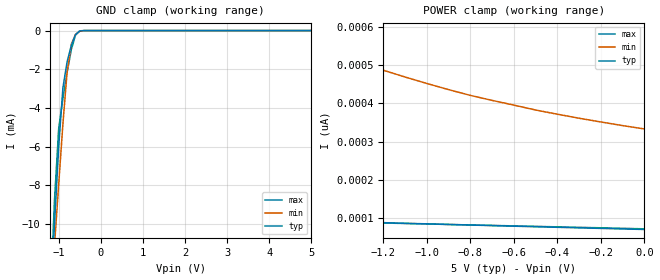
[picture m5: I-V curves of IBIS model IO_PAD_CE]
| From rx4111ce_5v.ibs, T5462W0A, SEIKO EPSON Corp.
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[Model]   IO_PAD_CE
Model_type Input
Enable Active-High
Polarity Non-Inverting
Vinh=4.4
Vinl=0.9
C_comp   2.5p   2.0p   3.0p
[Temperature Range] 25   105   -40
[Voltage Range]   5.0   4.5   5.5
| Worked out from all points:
|   GND clamp passes 1 mA (typ) near -0.73 V on its own axis
[GND Clamp]
-5V       -174.8mA   -140.3mA   -216.1mA
-1.2V     -14.09mA   -14.29mA   -13.9mA
-1.1V     -10.01mA   -11.11mA   -8.777mA
-1V       -6.002mA   -7.943mA   -5.058mA
-900mV    -2.958mA   -4.822mA   -3.504mA
-800mV    -1.61mA    -2.135mA   -2.158mA
-700mV    -762.7uA   -702uA     -983.6uA
-600mV    -207.8uA   -197.3uA   -229uA
-500mV    -21.89uA   -34.52uA   -13.51uA
-300mV    -47.04nA   -340.8nA   -3.548nA
5V        70.61pA    382.6pA    65.9pA
[POWER Clamp]
-5V       187.8pA    2.764nA    8.229uA
-4.7V     176.4pA    2.416nA    4.065nA
-4.6V     173.6pA    2.307nA    175.4pA
-4.5V     168.4pA    2.204nA    132.9pA
-3.7V     141.7pA    1.513nA    122.6pA
-3.1V     126.2pA    1.133nA    115pA
-1.7V     97.95pA    594.4pA    95.44pA
-1.6V     96.39pA    569.7pA    94.2pA
-1.2V     88.42pA    486.4pA    87.48pA
-800mV    82.21pA    420.8pA    82.47pA
-400mV    76.31pA    371.6pA    77.45pA
0V        70.62pA    333.2pA    72.33pA
